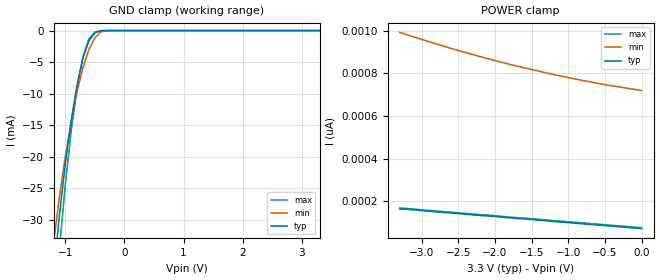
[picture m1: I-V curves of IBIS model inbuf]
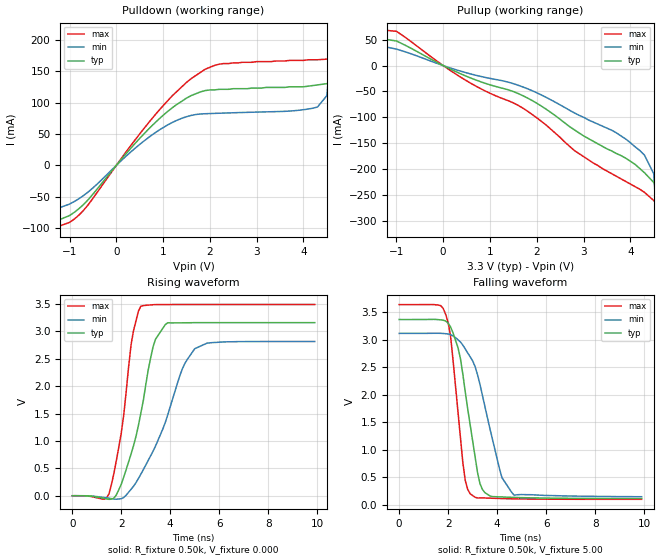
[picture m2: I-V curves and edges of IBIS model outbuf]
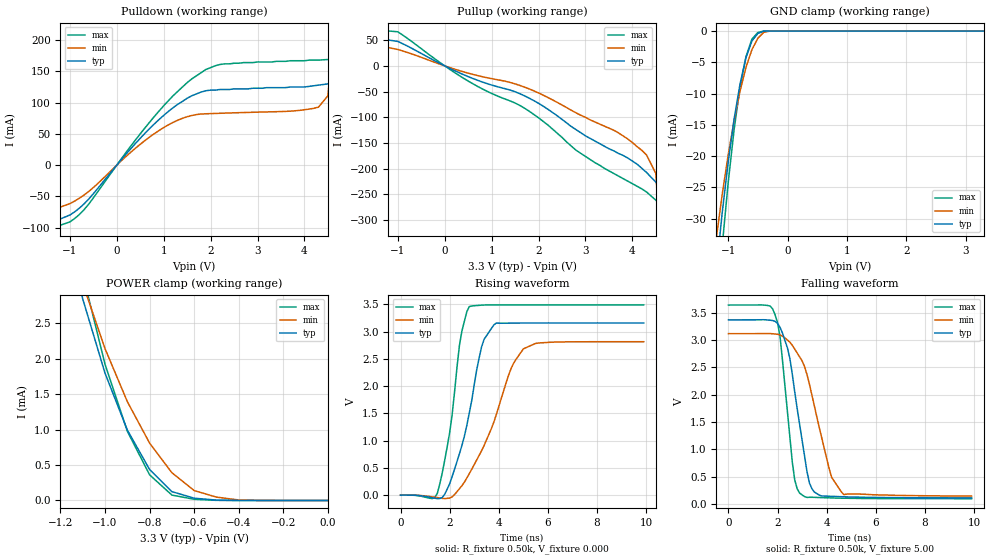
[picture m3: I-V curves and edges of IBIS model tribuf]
| IBIS file 43915n.ibs created by s2ibis2 version 1.0
| North Carolina State University Electronics Research Laboratory  1995
[IBIS ver]   2.1
[File name]   43915n.ibs
[File Rev]   0.1
[Date]   Wednesday, April 16, 1997
[Source]   IDT
[Notes]   1. Temp typ=25C, min=100C, max=0C 2. Ramp rates based on 500
   ohm load
[Copyright]   Copyright 1997, Integrated Device Technology, Inc.
[Disclaimer]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
|   Component IDT54/74FCT388915T
[Component]   IDT54/74FCT388915T
[Manufacturer]   Integrated Device Technology Inc.
[Package]
| Following package parameters are for SO28-7(SSOP) packages
| variable   typ   min   max
R_pkg   20.00m   15.00m   25.00m
L_pkg   3.10nH   2.00nH   4.20nH
C_pkg   0.30pF   0.26pF   0.34pF
[Pin]  signal_name   model_name   R_pin   L_pin   C_pin
1   GND   GND
2   Q5B   tribuf
3   VCC   POWER
4   OE/RSTB   inbuf
5   FEEDBACK   inbuf
6   REF_SEL   inbuf
7   SYNC(0)   inbuf
8   VCC(AN)   POWER
9   LF   inbuf
10   GND(AN)   GND
11   SYNC(1)   inbuf
12   FREQ_SEL   inbuf
13   GND   GND
14   Q0   tribuf
15   VCC   POWER
16   Q1   tribuf
17   GND   GND
18   PLL_EN   inbuf
19   LOCK   outbuf
20   GND   GND
21   Q2   tribuf
22   VCC   POWER
23   Q3   tribuf
24   GND   GND
25   Q/2   tribuf
26   2Q   tribuf
27   VCC   POWER
28   Q4   tribuf
| Models and submodels in the file (3): inbuf (Input), outbuf (Output), tribuf (3-state)
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| in   IN1   dummy_model
| oe   OE1   dummy_model
|   Model inbuf
[Model]   inbuf
Model_type   Input
Vinl =  0.800V
Vinh =  2.000V
C_comp   3.00pF   NA   NA
[Temperature Range]   25.00   100.00   0.000
[Voltage Range]   3.30V   3.00V   3.60V
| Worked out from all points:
|   GND clamp passes 1 mA (typ) near -0.55 V on its own axis
[GND_clamp]
| voltage   I(typ)   I(min)   I(max)
-3.3V     -45.02A    -40.87A    -46.46A
-1.2V     -38.87mA   -33.72mA   -46.57mA
-1.1V     -29.25mA   -26.32mA   -34.56mA
-1V       -21.08mA   -19.93mA   -24.38mA
-900mV    -14.13mA   -14.36mA   -15.81mA
-800mV    -8.469mA   -9.622mA   -8.979mA
-700mV    -4.247mA   -5.798mA   -4.09mA
-600mV    -1.585mA   -2.977mA   -1.278mA
-500mV    -389uA     -1.149mA   -232uA
-400mV    -20.6uA    -203uA     -9.215uA
-300mV    -264nA     -8.345uA   -70.34nA
3.3V      71.44pA    736pA      67.41pA
[POWER_clamp]
| voltage   I(typ)   I(min)   I(max)
-3.3V     164pA      992pA      168pA
-3.2V     162pA      981pA      166pA
-2.7V     147pA      927pA      151pA
-2.2V     133pA      878pA      137pA
-1.8V     122pA      842pA      126pA
-1.2V     105pA      794pA      109pA
-800mV    93.94pA    766pA      98.22pA
-400mV    82.69pA    741pA      86.97pA
0V        71.43pA    719pA      75.81pA
|   Model outbuf
[Model]   outbuf
Model_type   Output
Polarity   Non-Inverting
Vinl =  0.800V
Vinh =  2.000V
C_comp   3.00pF   NA   NA
[Temperature Range]   25.00   100.00   0.000
[Voltage Range]   3.30V   3.00V   3.60V
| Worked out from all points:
|   slope of the pulldown table from 0 to 0.495 V, typ, clamps not added: 11.6 ohm
|   slope of the pullup table from 0 to 0.495 V, typ, clamps not added: 24 ohm
|   rising waveform, R_fixture 0.50k, V_fixture 0.000: 20-80 % time 896ps typ, 1.44ns min, 593ps max; typ from 0 V to 3.16 V
|   falling waveform, R_fixture 0.50k, V_fixture 5.00: 20-80 % time 666ps typ, 959ps min, 461ps max; typ from 3.37 V to 0.109 V
[Pulldown]
| voltage   I(typ)   I(min)   I(max)
-3.3V     -50mA      -20mA      -70mA
-2.5V     -82mA      -60mA      -92mA
-1.5V     -95.1mA    -74.97mA   -104mA
-800mV    -68.95mA   -53.03mA   -79.14mA
900mV     72.89mA    55.4mA     86.45mA
1.9V      119mA      82.16mA    153mA
4.3V      128mA      92.85mA    168mA
4.5V      130mA      111mA      169mA
4.7V      141mA      276mA      172mA
4.9V      298mA      720mA      177mA
5.1V      776mA      1.302A     244mA
6.6V      5.909A     6.456A     5.041A
[Pullup]
| voltage   I(typ)   I(min)   I(max)
-3.3V     2mA        2mA        3mA
-1.9V     12.2mA     13.6mA     14mA
-1.7V     24.4mA     27.3mA     28.1mA
-1.5V     54.47mA    40.98mA    70.32mA
-1V       47.47mA    31.84mA    66.21mA
1.8V      -62.71mA   -44.77mA   -88.1mA
3.9V      -179mA     -142mA     -224mA
4.3V      -207mA     -173mA     -245mA
4.5V      -226mA     -209mA     -261mA
4.7V      -256mA     -496mA     -282mA
4.9V      -522mA     -1.594A    -307mA
6.6V      -16.85A    -18.41A    -14.25A
[Ramp]
| variable   typ   min   max
dV/dt_r   1.89/0.90n   1.69/1.44n   2.09/0.59n
dV/dt_f   1.94/0.67n   1.75/0.92n   2.12/0.46n
R_load = 0.50k
[Rising Waveform]
R_fixture = 0.50k
V_fixture = 0.000
| time   V(typ)   V(min)   V(max)
0s        0V         0V         0V
1.5ns     -65.43mV   -45.34mV   34.72mV
2ns       210mV      -54.62mV   1.145V
2.4ns     761mV      118mV      2.752V
2.8ns     1.508V     394mV      3.459V
3.4ns     2.856V     908mV      3.487V
3.9ns     3.156V     1.478V     3.488V
4.5ns     3.155V     2.32V      3.489V
5ns       3.158V     2.682V     3.489V
9.9ns     3.158V     2.814V     3.489V
[Falling Waveform]
R_fixture = 0.50k
V_fixture = 5.00
| time   V(typ)   V(min)   V(max)
0s        3.37V      3.117V     3.641V
1.9ns     3.342V     3.111V     3.463V
2.1ns     3.233V     3.093V     3.065V
2.4ns     2.86V      3.001V     1.697V
2.7ns     2.048V     2.833V     436mV
2.9ns     1.451V     2.69V      196mV
3.4ns     275mV      1.988V     120mV
4.2ns     138mV      487mV      108mV
4.7ns     129mV      169mV      103mV
9.9ns     109mV      142mV      94.33mV
|   Model tribuf
[Model]   tribuf
Model_type   3-state
Polarity   Non-Inverting
Enable   Active-High
Vinl =  0.800V
Vinh =  2.000V
C_comp   3.00pF   NA   NA
[Temperature Range]   25.00   100.00   0.000
[Voltage Range]   3.30V   3.00V   3.60V
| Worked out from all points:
|   slope of the pulldown table from 0 to 0.495 V, typ, clamps not added: 11.6 ohm
|   slope of the pullup table from 0 to 0.495 V, typ, clamps not added: 24 ohm
|   GND clamp passes 1 mA (typ) near -0.55 V on its own axis
|   POWER clamp passes 1 mA (typ) near -0.90 V on its own axis
|   rising waveform, R_fixture 0.50k, V_fixture 0.000: 20-80 % time 896ps typ, 1.44ns min, 593ps max; typ from 0 V to 3.16 V
|   falling waveform, R_fixture 0.50k, V_fixture 5.00: 20-80 % time 666ps typ, 959ps min, 461ps max; typ from 3.37 V to 0.109 V
[Pulldown]
| voltage   I(typ)   I(min)   I(max)
-3.3V     -50mA      -20mA      -70mA
-2.5V     -82mA      -60mA      -92mA
-1.5V     -95.1mA    -74.97mA   -104mA
-800mV    -68.95mA   -53.03mA   -79.14mA
900mV     72.89mA    55.4mA     86.45mA
1.9V      119mA      82.16mA    153mA
4.3V      128mA      92.85mA    168mA
4.5V      130mA      111mA      169mA
4.7V      141mA      276mA      172mA
4.9V      298mA      720mA      177mA
5.1V      776mA      1.302A     244mA
6.6V      5.909A     6.456A     5.041A
[Pullup]
| voltage   I(typ)   I(min)   I(max)
-3.3V     2mA        2mA        3mA
-1.9V     12.2mA     13.6mA     14mA
-1.7V     24.4mA     27.3mA     28.1mA
-1.5V     54.47mA    40.98mA    70.32mA
-1V       47.47mA    31.84mA    66.21mA
1.8V      -62.71mA   -44.77mA   -88.1mA
3.9V      -179mA     -142mA     -224mA
4.3V      -207mA     -173mA     -245mA
4.5V      -226mA     -209mA     -261mA
4.7V      -256mA     -496mA     -282mA
4.9V      -522mA     -1.594A    -307mA
6.6V      -16.85A    -18.41A    -14.25A
[GND_clamp]
| voltage   I(typ)   I(min)   I(max)
-3.3V     -16.77A    -15.21A    -17.33A
-1.2V     -38.28mA   -33.17mA   -45.9mA
-1.1V     -29.05mA   -26.11mA   -34.33mA
-1V       -21mA      -19.84mA   -24.28mA
-900mV    -14.09mA   -14.31mA   -15.76mA
-800mV    -8.456mA   -9.602mA   -8.965mA
-700mV    -4.244mA   -5.791mA   -4.087mA
-600mV    -1.584mA   -2.975mA   -1.277mA
-500mV    -389uA     -1.149mA   -232uA
-400mV    -20.55uA   -201uA     -9.204uA
-300mV    -264nA     -8.342uA   -70.38nA
3.3V      71.46pA    771nA      63.47pA
[POWER_clamp]
| voltage   I(typ)   I(min)   I(max)
-3.3V     5.777A     5.299A     5.941A
-1.1V     2.845mA    3.062mA    3.196mA
-1V       1.797mA    2.143mA    1.923mA
-900mV    995uA      1.396mA    978uA
-800mV    437uA      810uA      362uA
-700mV    125uA      392uA      76.41uA
-600mV    32.5uA     140uA      17.05uA
-500mV    5.486uA    47.49uA    1.9uA
-400mV    289nA      7.563uA    73.06nA
0V        71.43pA    719pA      75.83pA
[Ramp]
| variable   typ   min   max
dV/dt_r   1.89/0.90n   1.69/1.44n   2.09/0.59n
dV/dt_f   1.94/0.67n   1.75/0.92n   2.12/0.46n
R_load = 0.50k
[Rising Waveform]
R_fixture = 0.50k
V_fixture = 0.000
| time   V(typ)   V(min)   V(max)
0s        0V         0V         0V
1.5ns     -65.43mV   -45.34mV   34.72mV
2ns       210mV      -54.62mV   1.145V
2.4ns     761mV      118mV      2.752V
2.8ns     1.508V     394mV      3.459V
3.4ns     2.856V     908mV      3.487V
3.9ns     3.156V     1.478V     3.488V
4.5ns     3.155V     2.32V      3.489V
5ns       3.158V     2.682V     3.489V
9.9ns     3.158V     2.814V     3.489V
[Falling Waveform]
R_fixture = 0.50k
V_fixture = 5.00
| time   V(typ)   V(min)   V(max)
0s        3.37V      3.117V     3.641V
1.9ns     3.342V     3.111V     3.463V
2.1ns     3.233V     3.093V     3.065V
2.4ns     2.86V      3.001V     1.697V
2.7ns     2.048V     2.833V     436mV
2.9ns     1.451V     2.69V      196mV
3.4ns     275mV      1.988V     120mV
4.2ns     138mV      487mV      108mV
4.7ns     129mV      169mV      103mV
9.9ns     109mV      142mV      94.33mV
